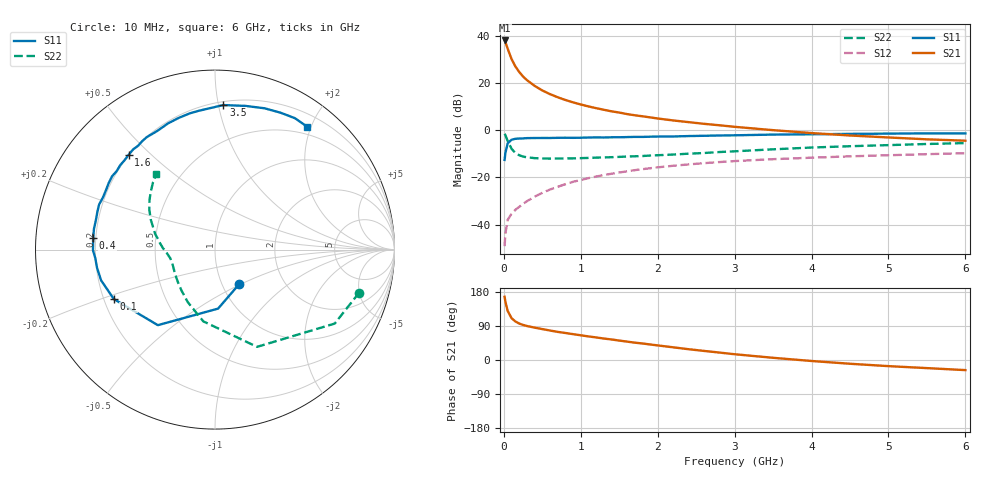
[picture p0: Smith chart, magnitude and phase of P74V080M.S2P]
! SIEMENS Small Signal Semiconductors
! BFP196
! Si NPN RF Bipolar Junction Transistor in SOT143
! VCE = 4 V  IC = 80 mA
! Common Emitter S-Parameters:  May  1996
# GHz  S  MA  R  50
!  f  S11  S21  S12  S22
! GHz  MAG  ANG  MAG  ANG  MAG  ANG  MAG  ANG
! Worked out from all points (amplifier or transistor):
!   36 points, 10 MHz to 6 GHz, reference 50 ohm
!   highest |S21| = 38.0 dB at 10 MHz (marker M1)
!   |S21| within 3 dB of that: start of sweep to 44.79 MHz
!   unconditionally stable (mu >= 1): 378 MHz to 4.435 GHz
!   at 250 MHz: K = 0.92, MSG = 27.0 dB, |S12| = -31.2 dB
!   at 1.4 GHz: K = 1.09, MAG = 11.4 dB, |S12| = -18.4 dB
!   at 6 GHz: K = 0.99, MSG = 2.7 dB, |S12| = -9.8 dB
!   S11 on the Smith chart (normalised r, x): 10 MHz: 1.20, -0.49; 100 MHz: 0.24, -0.22; 400 MHz: 0.19, +0.05; 1.6 GHz: 0.20, +0.43; 3.5 GHz: 0.22, +1.03; 6 GHz: 0.38, +1.94
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0.01  0.2347 -54.8  79.39 166.8  0.0035 78.9  0.8385 -16.6
0.02  0.3292 -87.0  73.49 154.0  0.0065 67.4  0.7841 -31.7
0.05  0.5279 -127.1  53.12 129.4  0.0126 54.6  0.5903 -66.6
0.1  0.6272 -153.9  32.12 110.5  0.017 50.6  0.405 -99.3
0.15  0.6574 -164.9  22.37 101.6  0.0206 52.4  0.3293 -117.5
0.2  0.665 -171.2  17.08 96.2  0.0238 56.2  0.2948 -129.3
0.25  0.6685 -175.9  13.69 92.5  0.0275 58.6  0.276 -138.1
0.3  0.6799 -179.7  11.48 89.7  0.0313 61.6  0.2664 -143.9
0.4  0.6816 174.5  8.674 85.4  0.0391 63.9  0.2561 -152.3
0.5  0.6842 170.3  6.945 81.6  0.0471 64.9  0.2516 -157.9
0.6  0.6838 166.0  5.793 77.8  0.0553 65.6  0.2504 -161.5
0.7  0.6885 162.0  4.981 74.2  0.0633 65.2  0.2511 -164.3
0.9  0.6886 154.9  3.88 68.2  0.0807 63.7  0.253 -168.6
1.1  0.6986 148.0  3.185 62.2  0.0965 61.6  0.2589 -171.6
1.3  0.7009 141.4  2.704 56.6  0.1123 59.0  0.2649 -174.3
1.6  0.7143 132.4  2.194 48.6  0.1345 54.7  0.2763 -177.9
2.2  0.7355 115.8  1.608 33.5  0.1763 45.6  0.3046 174.3
2.8  0.7718 100.6  1.272 19.7  0.2112 36.5  0.3445 165.3
3.5  0.8066 86.7  1.001 5.8  0.2432 26.4  0.3934 155.2
4.5  0.8345 70.6  0.772 -9.9  0.2794 14.3  0.4576 142.9
5.5  0.857 58.7  0.64 -21.4  0.3108 3.5  0.5099 132.6
6  0.8557 53.2  0.599 -26.7  0.3253 -2.2  0.5335 127.7
